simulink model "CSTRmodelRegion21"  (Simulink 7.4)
settings: Solver=ode15s  StartTime=0.0  StopTime=Tend  RelTol=1e-6
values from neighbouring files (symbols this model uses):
  cain = 2    [runDynSim321.m]    (also in sf_CSTR.m = cInVec(1))
  cbin = 1.5    [runDynSim321.m]    (also in sf_CSTR.m = cInVec(2))
undefined symbols (not defined in the file or in its folder): Floor, Ideal, internal, PI, Region2ControllerInitialValues, sigbuilder_block, Tdist, TimerScript, Tuninpars
libraries: simulink_extras x2

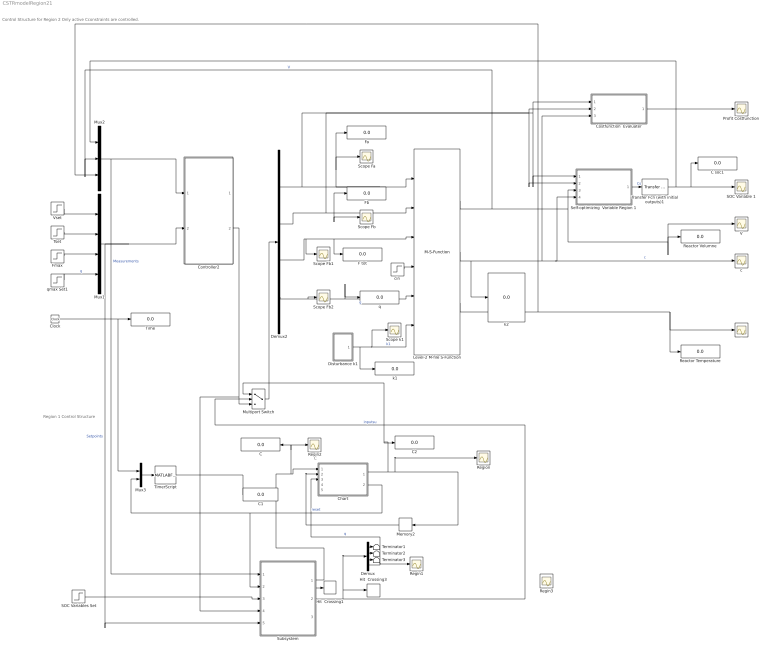
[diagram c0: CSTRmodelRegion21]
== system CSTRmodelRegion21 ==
  note: Control Structure for Region 2 Only active Cconstraints are controlled.
  note: Region 1 Control Structure
  note: C
  C : Display
  C soc1 : Display
  C1 : Display
  C2 : Display
  Chart : Stateflow chart
  Clock : Clock
  Controller2 : Subsystem
  Costfunction  Evaluater : Subsystem
  Demux : Demux
  Demux2 : Demux
  Disturbance k1 : Subsystem
  F tot : Display
  Fa : Display
  Fb : Display
  Fmax : Step  Time=0  Before=22  After=22  SampleTime=0
  Hit  Crossing1 : HitCross  HitCrossingOffset=1000  HitCrossingDirection=falling
  Hit  Crossing3 : HitCross  HitCrossingOffset=1000  HitCrossingDirection=rising
  Level-2 M-file S-Function : M-S-Function  FunctionName=sf_CSTR
  Memory2 : Memory  X0=1
  Multiport Switch : MultiPortSwitch  Inputs=2  OutDataType=fixdt(1, 16)  OutScaling=2^0
  Mux1 : Mux
  Mux2 : Mux  Inputs=3
  Mux3 : Mux  Inputs=2
  Profit Costfunction : Scope
  Reactor Temperature : Display
  Reactor Volumne : Display
  Regin1 : Scope
  Regin2 : Scope
  Regin3 : Scope
  Region : Scope
  SOC Variable 1 : Scope
  SOC Variables Set : Step  Time=0  After=0  SampleTime=0
  Scope Fa : Scope
  Scope Fb : Scope
  Scope Fb1 : Scope
  Scope Fb2 : Scope
  Scope k1 : Scope
  Self-optimizing  Variable Region 1 : Stateflow chart
  Subsystem : Subsystem
  T : Scope
  Terminator1 : Terminator
  Terminator2 : Terminator
  Terminator3 : Terminator
  Time : Display
  TimerScript : MATLABFcn  MATLABFcn=TimerScript(u(1),u(2))
  Transfer Fcn (with initial outputs)1 : simulink_extras/Additional Linear/Transfer Fcn (with initial outputs)  SystemSampleTime=-1  N=[1]  D="[1  1]"  Y0=41  U0=0
  Tset : Step  Time=250  Before=350  After=350  SampleTime=0
  V : Scope
  Vset : Step  Time=0  Before=500  After=500  SampleTime=0
  c : Scope
  cin : Step  Time=0  Before=[cain cbin 0 0]  After=[cain cbin 0 0]  SampleTime=0
  k1 : Display
  k2 : Display
  q : Display
  qmax Set1 : Step  Time=0  Before=1000  After=1000  SampleTime=0
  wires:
  cin/1 -> Level-2 M-file S-Function/4
  Level-2 M-file S-Function/1 -> Mux2/2, Self-optimizing  Variable Region 1/3(V), V/1, Reactor Volumne/1  "V"
  Level-2 M-file S-Function/2 -> Costfunction  Evaluater/3(Concentrations), c/1, Self-optimizing  Variable Region 1/4(cVector), k2/1  "c"
  Level-2 M-file S-Function/3 -> T/1, Reactor Temperature/1, Mux2/3  "T"
  Costfunction  Evaluater/1(Objective) -> Profit Costfunction/1
  Self-optimizing  Variable Region 1/1(cs) -> Transfer Fcn (with initial outputs)1/1  "Cs"
  Disturbance k1/1(Out1) -> Scope k1/1, Level-2 M-file S-Function/6, k1/1  "k1"
  Clock/1 -> Time/1, Mux3/1
  qmax Set1/1 -> Mux1/4  "q"
  Vset/1 -> Mux1/1
  Fmax/1 -> Mux1/3
  Tset/1 -> Mux1/2
  Mux2/1 -> Controller2/1(In1), Subsystem/1(In1)  "Measurements"
  Demux2/1 -> Costfunction  Evaluater/1(Fa), Self-optimizing  Variable Region 1/1(Fa), Level-2 M-file S-Function/1, Fa/1, Scope Fa/1
  Demux2/2 -> Costfunction  Evaluater/2(Fb), Self-optimizing  Variable Region 1/2(Fb), Scope Fb/1, Level-2 M-file S-Function/2, Fb/1
  Demux2/3 -> Level-2 M-file S-Function/3, F tot/1, Scope Fb1/1
  Demux2/4 -> Level-2 M-file S-Function/5, q/1, Scope Fb2/1  "q"
  Mux1/1 -> Controller2/2(In2), Subsystem/5(In5)  "Setpoints"
  Controller2/2(Out6) -> Multiport Switch/3, Subsystem/4(In4)
  SOC Variables Set/1 -> Subsystem/3(In3)
  Chart/2(reset) -> Subsystem/2(In2), Mux3/2  "reset"
  Multiport Switch/1 -> Demux2/1
  Subsystem/2(Out2) -> Hit  Crossing3/1, Demux/1, Multiport Switch/2  "inputsu"
  Transfer Fcn (with initial outputs)1/1 -> Mux2/1, SOC Variable 1/1, C soc1/1
  Subsystem/1(Out1) -> Chart/1(c1), C/1, Regin2/1, Hit  Crossing1/1
  Mux3/1 -> TimerScript/1
  TimerScript/1 -> C1/1
  Memory2/1 -> Chart/2(r)
  Demux/1 -> Terminator1/1
  Demux/2 -> Terminator2/1
  Demux/3 -> Terminator3/1
  Demux/4 -> Chart/3(q), Regin1/1  "q"
  Chart/1(R) -> Region/1, Memory2/1, C2/1, Multiport Switch/1

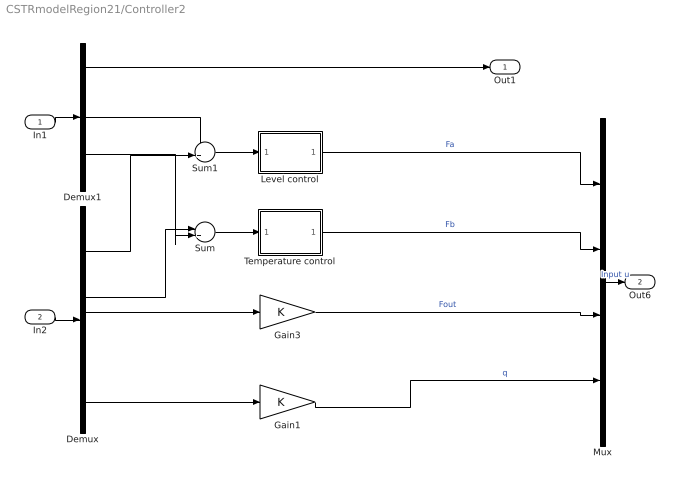
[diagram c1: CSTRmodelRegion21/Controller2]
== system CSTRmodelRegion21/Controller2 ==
  In1 : Inport
  In2 : Inport  Port=2
  Demux : Demux
  Demux1 : Demux  Outputs=3
  Gain1 : Gain  ParameterDataType=fixdt(1, 16)  ParameterScaling=2^0  OutDataType=fixdt(1, 16)  OutScaling=2^0
  Gain3 : Gain  ParameterDataType=fixdt(1, 16)  ParameterScaling=2^0  OutDataType=fixdt(1, 16)  OutScaling=2^0
  Level control : Subsystem  AncestorBlock=simulink/Continuous/PID Controller  DialogController=pidpack.PIDConfig.pidDDGCreate  DialogControllerArgs=DataTag0  mask(PID 1dof){Controller=PI, TimeDomain=Continuous-time, SampleTime=1, IntegratorMethod=Forward Euler, FilterMethod=Forward Euler, Form=Ideal, P=35*2, I=0.024, D=0, N=100, InitialConditionSource=internal, InitialConditionForIntegrator=Region2ControllerInitialValues.Level, InitialConditionForFilter=0, ExternalReset=none, IgnoreLimit=off, ZeroCross=on, LimitOutput=on, UpperSaturationLimit=10, LowerSaturationLimit=4, LinearizeAsGain=off, AntiWindupMode=back-calculation, Kb=1, TrackingMode=off, Kt=1, RndMeth=Floor, SaturateOnIntegerOverflow=off, LockScale=off, PParamMin=[], PParamMax=[], PParamDataTypeStr=Inherit: Inherit via internal rule, IParamMin=[], IParamMax=[], IParamDataTypeStr=Inherit: Inherit via internal rule, DParamMin=[], DParamMax=[], DParamDataTypeStr=Inherit: Inherit via internal rule, NParamMin=[], NParamMax=[], NParamDataTypeStr=Inherit: Inherit via internal rule, KbParamMin=[], KbParamMax=[], KbParamDataTypeStr=Inherit: Inherit via internal rule, KtParamMin=[], KtParamMax=[], KtParamDataTypeStr=Inherit: Inherit via internal rule, POutMin=[], POutMax=[], POutDataTypeStr=Inherit: Inherit via internal rule, IOutMin=[], IOutMax=[], IOutDataTypeStr=Inherit: Inherit via internal rule, DOutMin=[], DOutMax=[], DOutDataTypeStr=Inherit: Inherit via internal rule, NOutMin=[], NOutMax=[], NOutDataTypeStr=Inherit: Inherit via internal rule, KbOutMin=[], KbOutMax=[], KbOutDataTypeStr=Inherit: Inherit via internal rule, KtOutMin=[], KtOutMax=[], KtOutDataTypeStr=Inherit: Inherit via internal rule, IntegratorOutMin=[], IntegratorOutMax=[], IntegratorOutDataTypeStr=Inherit: Inherit via internal rule, FilterOutMin=[], FilterOutMax=[], FilterOutDataTypeStr=Inherit: Inherit via internal rule, SumOutMin=[], SumOutMax=[], SumOutDataTypeStr=Inherit: Inherit via internal rule, SumI1OutMin=[], SumI1OutMax=[], SumI1OutDataTypeStr=Inherit: Inherit via internal rule, SumI2OutMin=[], SumI2OutMax=[], SumI2OutDataTypeStr=Inherit: Inherit via internal rule, SumI3OutMin=[], SumI3OutMax=[], SumI3OutDataTypeStr=Inherit: Inherit via internal rule, SumDOutMin=[], SumDOutMax=[], SumDOutDataTypeStr=Inherit: Inherit via internal rule, SumAccumDataTypeStr=Inherit: Inherit via internal rule, SumI1AccumDataTypeStr=Inherit: Inherit via internal rule, SumI2AccumDataTypeStr=Inherit: Inherit via internal rule, SumI3AccumDataTypeStr=Inherit: Inherit via internal rule, SumDAccumDataTypeStr=Inherit: Inherit via internal rule, SaturationOutMin=[], SaturationOutMax=[], SaturationOutDataTypeStr=Inherit: Same as input, IntegratorContinuousStateAttributes='', IntegratorStateIdentifier=, IntegratorStateMustResolveToSignalObject=off, IntegratorRTWStateStorageClass=Auto, IntegratorRTWStateStorageTypeQualifier=, FilterContinuousStateAttributes='', FilterStateIdentifier=, FilterStateMustResolveToSignalObject=off, FilterRTWStateStorageClass=Auto, FilterRTWStateStorageTypeQualifier=}
      mask prompts: TimeDomain "Time-domain:"; SampleTime "Sample time (-1 for inherited):"; IntegratorMethod "Integrator method:"; FilterMethod "Filter method:"; Form "Controller form:"; P "Proportional (P):"; I "Integral (I):"; D "Derivative (D):"; N "Filter coefficient (N):"; InitialConditionSource "Source:"; InitialConditionForIntegrator "Integrator:"; InitialConditionForFilter "Filter:"; ExternalReset "External reset:"; IgnoreLimit "Ignore reset when linearizing"; ZeroCross "Enable zero-crossing detection"; LimitOutput "Limit output"; UpperSaturationLimit "Upper saturation limit:"; LowerSaturationLimit "Lower saturation limit:"; LinearizeAsGain "Ignore saturation when linearizing"; AntiWindupMode "Anti-windup method:"; Kb "Back-calculation coefficient (Kb):"; TrackingMode "Enable tracking mode"; Kt "Tracking coefficient (Kt):"; RndMeth "Integer rounding mode:"; SaturateOnIntegerOverflow "Saturate on integer overflow"; LockScale "Lock data type settings against changes by the fixed-point tools"; PParamMin "P parameter minimum:"; PParamMax "P parameter maximum:"; PParamDataTypeStr "P parameter:"; IParamMin "I parameter minimum:"; IParamMax "I parameter maximum:"; IParamDataTypeStr "I parameter:"; DParamMin "D parameter minimum:"; DParamMax "D parameter maximum:"; DParamDataTypeStr "D parameter:"; NParamMin "N parameter minimum:"; NParamMax "N parameter maximum:"; NParamDataTypeStr "N parameter:"; KbParamMin "Kb parameter minimum:"; KbParamMax "Kb parameter maximum:"; KbParamDataTypeStr "Kb parameter:"; KtParamMin "Kt parameter minimum:"; KtParamMax "Kt parameter maximum:"; KtParamDataTypeStr "Kt parameter:"; POutMin "P product output minimum:"; POutMax "P product output maximum:"; POutDataTypeStr "P product output:"; IOutMin "I product output minimum:"; IOutMax "I product output maximum:"; IOutDataTypeStr "I product output:"; DOutMin "D product output minimum:"; DOutMax "D product output maximum:"; DOutDataTypeStr "D product output:"; NOutMin "N product output minimum:"; NOutMax "N product output maximum:"; NOutDataTypeStr "N product output:"; KbOutMin "Kb product output minimum:"; KbOutMax "Kb product output maximum:"; KbOutDataTypeStr "Kb product output:"; KtOutMin "Kt product output minimum:"; KtOutMax "Kt product output maximum:"; KtOutDataTypeStr "Kt product output:"; IntegratorOutMin "Integrator output minimum:"; IntegratorOutMax "Integrator output maximum:"; IntegratorOutDataTypeStr "Integrator output:"; FilterOutMin "Filter output minimum:"; FilterOutMax "Filter output maximum:"; FilterOutDataTypeStr "Filter output:"; SumOutMin "Sum output minimum:"; SumOutMax "Sum output maximum:"; SumOutDataTypeStr "Sum output:"; SumI1OutMin "SumI1 output minimum:"; SumI1OutMax "SumI1 output maximum:"; SumI1OutDataTypeStr "SumI1 output:"; SumI2OutMin "SumI2 output minimum:"; SumI2OutMax "SumI2 output maximum:"; SumI2OutDataTypeStr "SumI2 output:"; SumI3OutMin "SumI3 output minimum:"; SumI3OutMax "SumI3 output maximum:"; SumI3OutDataTypeStr "SumI3 output:"; SumDOutMin "SumD output minimum:"; SumDOutMax "SumD output maximum:"; SumDOutDataTypeStr "SumD output:"; SumAccumDataTypeStr "Accumulator of Sum:"; SumI1AccumDataTypeStr "Accumulator of SumI1:"; SumI2AccumDataTypeStr "Accumulator of SumI2:"; SumI3AccumDataTypeStr "Accumulator of SumI3:"; SumDAccumDataTypeStr "Accumulator of SumD:"; SaturationOutMin "Saturation output minimum:"; SaturationOutMax "Saturation output maximum:"; SaturationOutDataTypeStr "Saturation output:"; IntegratorContinuousStateAttributes "State name: (e.g., 'position')"; IntegratorStateIdentifier "State name:"; IntegratorStateMustResolveToSignalObject "State name must resolve to Simulink signal object"; IntegratorRTWStateStorageClass "Real-Time Workshop storage class:"; IntegratorRTWStateStorageTypeQualifier "Real-Time Workshop storage type qualifier:"; FilterContinuousStateAttributes "State name: (e.g., 'position')"; FilterStateIdentifier "State name:"; FilterStateMustResolveToSignalObject "State name must resolve to Simulink signal object"; FilterRTWStateStorageClass "Real-Time Workshop storage class:"; FilterRTWStateStorageTypeQualifier "Real-Time Workshop storage type qualifier:"
      mask help: This block implements continuous- and discrete-time PID control algorithms and includes advanced features such as anti-windup, external reset, and signal tracking. You can tune the PID gains automatically using the 'Tune...' button (requires Simulink Control Design).
      mask init:
      | [shiftx shifty satshiftx satshifty] = pidpack.PIDConfig.configPID(gcbh);
  Mux : Mux
  Sum : Sum  Inputs=|+-  OutDataType=fixdt(1, 16)  OutScaling=2^0
  Sum1 : Sum  Inputs=-+|  OutDataType=fixdt(1, 16)  OutScaling=2^0
  Temperature control : Subsystem  AncestorBlock=simulink/Continuous/PID Controller  DialogController=pidpack.PIDConfig.pidDDGCreate  DialogControllerArgs=DataTag1  mask(PID 1dof){Controller=PI, TimeDomain=Continuous-time, SampleTime=1, IntegratorMethod=Forward Euler, FilterMethod=Forward Euler, Form=Ideal, P=-0.845/2/5, I=1, D=0, N=100, InitialConditionSource=internal, InitialConditionForIntegrator=Region2ControllerInitialValues.Temperature, InitialConditionForFilter=0, ExternalReset=none, IgnoreLimit=off, ZeroCross=on, LimitOutput=on, UpperSaturationLimit=1e3, LowerSaturationLimit=10, LinearizeAsGain=off, AntiWindupMode=back-calculation, Kb=1, TrackingMode=off, Kt=1, RndMeth=Floor, SaturateOnIntegerOverflow=off, LockScale=off, PParamMin=[], PParamMax=[], PParamDataTypeStr=Inherit: Inherit via internal rule, IParamMin=[], IParamMax=[], IParamDataTypeStr=Inherit: Inherit via internal rule, DParamMin=[], DParamMax=[], DParamDataTypeStr=Inherit: Inherit via internal rule, NParamMin=[], NParamMax=[], NParamDataTypeStr=Inherit: Inherit via internal rule, KbParamMin=[], KbParamMax=[], KbParamDataTypeStr=Inherit: Inherit via internal rule, KtParamMin=[], KtParamMax=[], KtParamDataTypeStr=Inherit: Inherit via internal rule, POutMin=[], POutMax=[], POutDataTypeStr=Inherit: Inherit via internal rule, IOutMin=[], IOutMax=[], IOutDataTypeStr=Inherit: Inherit via internal rule, DOutMin=[], DOutMax=[], DOutDataTypeStr=Inherit: Inherit via internal rule, NOutMin=[], NOutMax=[], NOutDataTypeStr=Inherit: Inherit via internal rule, KbOutMin=[], KbOutMax=[], KbOutDataTypeStr=Inherit: Inherit via internal rule, KtOutMin=[], KtOutMax=[], KtOutDataTypeStr=Inherit: Inherit via internal rule, IntegratorOutMin=[], IntegratorOutMax=[], IntegratorOutDataTypeStr=Inherit: Inherit via internal rule, FilterOutMin=[], FilterOutMax=[], FilterOutDataTypeStr=Inherit: Inherit via internal rule, SumOutMin=[], SumOutMax=[], SumOutDataTypeStr=Inherit: Inherit via internal rule, SumI1OutMin=[], SumI1OutMax=[], SumI1OutDataTypeStr=Inherit: Inherit via internal rule, SumI2OutMin=[], SumI2OutMax=[], SumI2OutDataTypeStr=Inherit: Inherit via internal rule, SumI3OutMin=[], SumI3OutMax=[], SumI3OutDataTypeStr=Inherit: Inherit via internal rule, SumDOutMin=[], SumDOutMax=[], SumDOutDataTypeStr=Inherit: Inherit via internal rule, SumAccumDataTypeStr=Inherit: Inherit via internal rule, SumI1AccumDataTypeStr=Inherit: Inherit via internal rule, SumI2AccumDataTypeStr=Inherit: Inherit via internal rule, SumI3AccumDataTypeStr=Inherit: Inherit via internal rule, SumDAccumDataTypeStr=Inherit: Inherit via internal rule, SaturationOutMin=[], SaturationOutMax=[], SaturationOutDataTypeStr=Inherit: Same as input, IntegratorContinuousStateAttributes='', IntegratorStateIdentifier=, IntegratorStateMustResolveToSignalObject=off, IntegratorRTWStateStorageClass=Auto, IntegratorRTWStateStorageTypeQualifier=, FilterContinuousStateAttributes='', FilterStateIdentifier=, FilterStateMustResolveToSignalObject=off, FilterRTWStateStorageClass=Auto, FilterRTWStateStorageTypeQualifier=}
      mask prompts: TimeDomain "Time-domain:"; SampleTime "Sample time (-1 for inherited):"; IntegratorMethod "Integrator method:"; FilterMethod "Filter method:"; Form "Controller form:"; P "Proportional (P):"; I "Integral (I):"; D "Derivative (D):"; N "Filter coefficient (N):"; InitialConditionSource "Source:"; InitialConditionForIntegrator "Integrator:"; InitialConditionForFilter "Filter:"; ExternalReset "External reset:"; IgnoreLimit "Ignore reset when linearizing"; ZeroCross "Enable zero-crossing detection"; LimitOutput "Limit output"; UpperSaturationLimit "Upper saturation limit:"; LowerSaturationLimit "Lower saturation limit:"; LinearizeAsGain "Ignore saturation when linearizing"; AntiWindupMode "Anti-windup method:"; Kb "Back-calculation coefficient (Kb):"; TrackingMode "Enable tracking mode"; Kt "Tracking coefficient (Kt):"; RndMeth "Integer rounding mode:"; SaturateOnIntegerOverflow "Saturate on integer overflow"; LockScale "Lock data type settings against changes by the fixed-point tools"; PParamMin "P parameter minimum:"; PParamMax "P parameter maximum:"; PParamDataTypeStr "P parameter:"; IParamMin "I parameter minimum:"; IParamMax "I parameter maximum:"; IParamDataTypeStr "I parameter:"; DParamMin "D parameter minimum:"; DParamMax "D parameter maximum:"; DParamDataTypeStr "D parameter:"; NParamMin "N parameter minimum:"; NParamMax "N parameter maximum:"; NParamDataTypeStr "N parameter:"; KbParamMin "Kb parameter minimum:"; KbParamMax "Kb parameter maximum:"; KbParamDataTypeStr "Kb parameter:"; KtParamMin "Kt parameter minimum:"; KtParamMax "Kt parameter maximum:"; KtParamDataTypeStr "Kt parameter:"; POutMin "P product output minimum:"; POutMax "P product output maximum:"; POutDataTypeStr "P product output:"; IOutMin "I product output minimum:"; IOutMax "I product output maximum:"; IOutDataTypeStr "I product output:"; DOutMin "D product output minimum:"; DOutMax "D product output maximum:"; DOutDataTypeStr "D product output:"; NOutMin "N product output minimum:"; NOutMax "N product output maximum:"; NOutDataTypeStr "N product output:"; KbOutMin "Kb product output minimum:"; KbOutMax "Kb product output maximum:"; KbOutDataTypeStr "Kb product output:"; KtOutMin "Kt product output minimum:"; KtOutMax "Kt product output maximum:"; KtOutDataTypeStr "Kt product output:"; IntegratorOutMin "Integrator output minimum:"; IntegratorOutMax "Integrator output maximum:"; IntegratorOutDataTypeStr "Integrator output:"; FilterOutMin "Filter output minimum:"; FilterOutMax "Filter output maximum:"; FilterOutDataTypeStr "Filter output:"; SumOutMin "Sum output minimum:"; SumOutMax "Sum output maximum:"; SumOutDataTypeStr "Sum output:"; SumI1OutMin "SumI1 output minimum:"; SumI1OutMax "SumI1 output maximum:"; SumI1OutDataTypeStr "SumI1 output:"; SumI2OutMin "SumI2 output minimum:"; SumI2OutMax "SumI2 output maximum:"; SumI2OutDataTypeStr "SumI2 output:"; SumI3OutMin "SumI3 output minimum:"; SumI3OutMax "SumI3 output maximum:"; SumI3OutDataTypeStr "SumI3 output:"; SumDOutMin "SumD output minimum:"; SumDOutMax "SumD output maximum:"; SumDOutDataTypeStr "SumD output:"; SumAccumDataTypeStr "Accumulator of Sum:"; SumI1AccumDataTypeStr "Accumulator of SumI1:"; SumI2AccumDataTypeStr "Accumulator of SumI2:"; SumI3AccumDataTypeStr "Accumulator of SumI3:"; SumDAccumDataTypeStr "Accumulator of SumD:"; SaturationOutMin "Saturation output minimum:"; SaturationOutMax "Saturation output maximum:"; SaturationOutDataTypeStr "Saturation output:"; IntegratorContinuousStateAttributes "State name: (e.g., 'position')"; IntegratorStateIdentifier "State name:"; IntegratorStateMustResolveToSignalObject "State name must resolve to Simulink signal object"; IntegratorRTWStateStorageClass "Real-Time Workshop storage class:"; IntegratorRTWStateStorageTypeQualifier "Real-Time Workshop storage type qualifier:"; FilterContinuousStateAttributes "State name: (e.g., 'position')"; FilterStateIdentifier "State name:"; FilterStateMustResolveToSignalObject "State name must resolve to Simulink signal object"; FilterRTWStateStorageClass "Real-Time Workshop storage class:"; FilterRTWStateStorageTypeQualifier "Real-Time Workshop storage type qualifier:"
      mask help: This block implements continuous- and discrete-time PID control algorithms and includes advanced features such as anti-windup, external reset, and signal tracking. You can tune the PID gains automatically using the 'Tune...' button (requires Simulink Control Design).
      mask init:
      | [shiftx shifty satshiftx satshifty] = pidpack.PIDConfig.configPID(gcbh);
  Out1 : Outport
  Out6 : Outport  Port=2
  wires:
  Sum/1 -> Temperature control/1(u)
  Sum1/1 -> Level control/1(u)
  Demux/1 -> Sum1/2
  Demux/2 -> Sum/1
  Demux/3 -> Gain3/1
  Demux/4 -> Gain1/1
  Demux1/2 -> Sum1/1
  Demux1/3 -> Sum/2
  Demux1/1 -> Out1/1
  In1/1 -> Demux1/1
  Level control/1(y) -> Mux/1  "Fa"
  Temperature control/1(y) -> Mux/2  "Fb"
  Gain3/1 -> Mux/3  "Fout"
  In2/1 -> Demux/1
  Gain1/1 -> Mux/4  "q"
  Mux/1 -> Out6/1  "Input u"

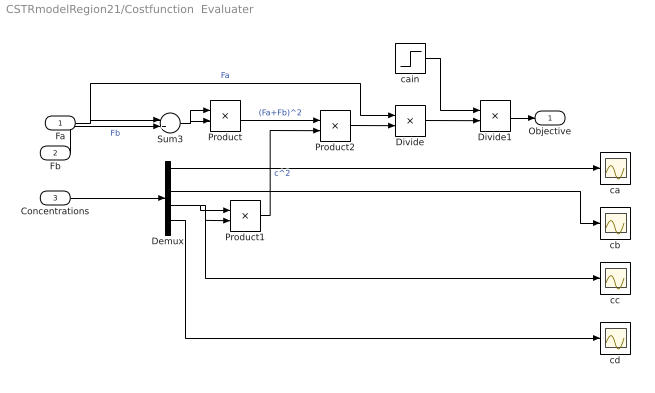
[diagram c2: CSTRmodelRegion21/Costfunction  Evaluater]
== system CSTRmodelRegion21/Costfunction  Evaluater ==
  Fa : Inport
  Fb : Inport  Port=2
  Concentrations : Inport  Port=3
  Demux : Demux
  Divide : Product  Inputs=/*  OutDataType=fixdt(1, 16)  OutScaling=2^-10
  Divide1 : Product  Inputs=/*  OutDataType=fixdt(1, 16)  OutScaling=2^-10
  Product : Product  OutDataType=fixdt(1, 16)  OutScaling=2^0
  Product1 : Product  OutDataType=fixdt(1, 16)  OutScaling=2^0
  Product2 : Product  OutDataType=fixdt(1, 16)  OutScaling=2^0
  Sum3 : Sum  Inputs=|++  OutDataType=fixdt(1, 16)  OutScaling=2^0
  ca : Scope
  cain : Step  Before=cain  After=cain  SampleTime=0
  cb : Scope
  cc : Scope
  cd : Scope
  Objective : Outport
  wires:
  Sum3/1 -> Product/1, Product/2
  Demux/3 -> Product1/1, Product1/2, cc/1
  Product/1 -> Product2/1  "(Fa+Fb)^2"
  Product1/1 -> Product2/2  "c^2"
  Product2/1 -> Divide/2
  Divide/1 -> Divide1/2
  cain/1 -> Divide1/1
  Fa/1 -> Sum3/1, Divide/1  "Fa"
  Fb/1 -> Sum3/2  "Fb"
  Concentrations/1 -> Demux/1
  Divide1/1 -> Objective/1
  Demux/1 -> ca/1
  Demux/2 -> cb/1
  Demux/4 -> cd/1

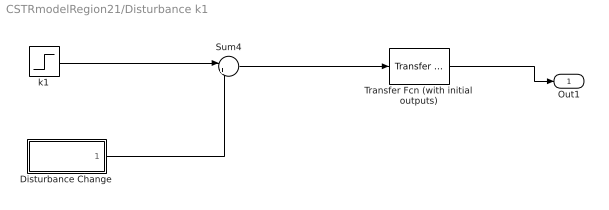
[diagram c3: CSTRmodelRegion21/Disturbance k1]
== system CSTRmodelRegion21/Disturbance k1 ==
  Disturbance Change : Subsystem  Tag=STV Subsys  LoadFcn=sigbuilder_block('load');  StartFcn=sigbuilder_block('start');  StopFcn=sigbuilder_block('stop');  ClipboardFcn=sigbuilder_block('clipboard');
  Sum4 : Sum  Inputs=|++  OutDataType=fixdt(1, 16)  OutScaling=2^0
  Transfer Fcn (with initial outputs) : simulink_extras/Additional Linear/Transfer Fcn (with initial outputs)  SystemSampleTime=-1  N=[1]  D="[50  1]"  Y0=0.75  U0=0
  k1 : Step  Time=Tdist  After=0  SampleTime=0
  Out1 : Outport
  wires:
  Sum4/1 -> Transfer Fcn (with initial outputs)/1
  Disturbance Change/1(Signal 1) -> Sum4/2
  k1/1 -> Sum4/1
  Transfer Fcn (with initial outputs)/1 -> Out1/1

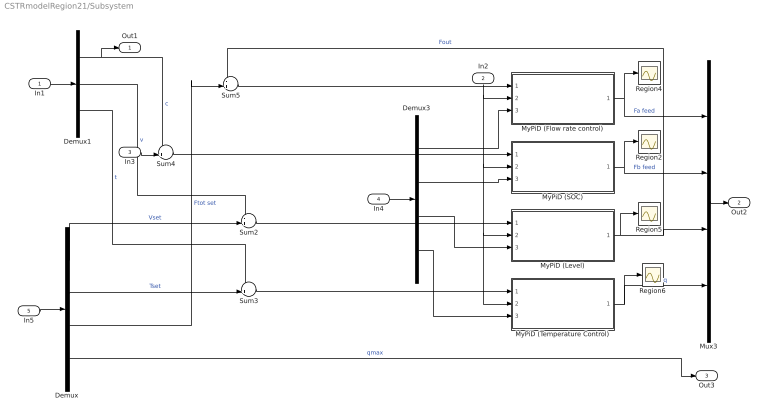
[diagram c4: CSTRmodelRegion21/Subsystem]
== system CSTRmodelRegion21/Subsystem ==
  In1 : Inport
  In2 : Inport  Port=2
  In3 : Inport  Port=3
  In4 : Inport  Port=4
  In5 : Inport  Port=5
  Demux : Demux
  Demux1 : Demux  Outputs=3
  Demux3 : Demux
  Mux3 : Mux
  MyPiD (Flow rate control) : Subsystem  mask{Kp=Tuninpars.Reg1.FlowController.Kp, TauiInv=Tuninpars.Reg1.FlowController.TauiInv, UB=[inf], LB=2}
      mask prompts: Kp "Proportional Gain Kp"; TauiInv "Inverse Integral time"; UB "Upper bound"; LB "Lower bound"
  MyPiD (Level) : Subsystem  mask{Kp=Tuninpars.Reg1.LevelController.Kp, TauiInv=Tuninpars.Reg1.LevelController.TauiInv, UB=[40], LB=2}
      mask prompts: Kp "Proportional Gain Kp"; TauiInv "Inverse Integral time"; UB "Upper bound"; LB "Lower bound"
  MyPiD (SOC) : Subsystem  mask{Kp=Tuninpars.Reg1.SocController.Kp, TauiInv=Tuninpars.Reg1.SocController.TauiInv, UB=inf, LB=2}
      mask prompts: Kp "Proportional Gain Kp"; TauiInv "Inverse Integral time"; UB "Upper bound"; LB "Lower bound"
  MyPiD (Temperature Control) : Subsystem  mask{Kp=Tuninpars.Reg1.TempController.Kp, TauiInv=Tuninpars.Reg1.TempController.TauiInv, UB=1000, LB=1}
      mask prompts: Kp "Proportional Gain Kp"; TauiInv "Inverse Integral time"; UB "Upper bound"; LB "Lower bound"
  Region{2,4..6} (4 alike) : Scope
  Sum{2..5} (4 alike) : Sum  Inputs=-+|  OutDataType=fixdt(1, 16)  OutScaling=2^0
  Out1 : Outport
  Out2 : Outport  Port=2
  Out3 : Outport  Port=3
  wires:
  Sum5/1 -> MyPiD (Flow rate control)/1(In1)
  Sum4/1 -> MyPiD (SOC)/1(In1)
  MyPiD (SOC)/1(Out1) -> Mux3/2, Region2/1  "Fb feed"
  Sum2/1 -> MyPiD (Level)/1(In1)
  MyPiD (Level)/1(Out1) -> Sum5/1, Mux3/3, Region5/1  "Fout"
  Sum3/1 -> MyPiD (Temperature Control)/1(In1)
  MyPiD (Temperature Control)/1(Out1) -> Region6/1, Mux3/4  "q"
  Demux1/1 -> Sum4/1, Out1/1  "c"
  Demux1/2 -> Sum2/1  "v"
  Demux1/3 -> Sum3/1  "t"
  Demux/3 -> Sum5/2  "Ftot set"
  MyPiD (Flow rate control)/1(Out1) -> Mux3/1, Region4/1  "Fa feed"
  Demux/2 -> Sum3/2  "Tset"
  Demux/1 -> Sum2/2  "Vset"
  Demux3/1 -> MyPiD (Flow rate control)/3(In3)
  Demux3/2 -> MyPiD (SOC)/3(In3)
  Demux3/3 -> MyPiD (Level)/3(In3)
  Demux3/4 -> MyPiD (Temperature Control)/3(In3)
  In1/1 -> Demux1/1
  In2/1 -> MyPiD (Flow rate control)/2(In2), MyPiD (SOC)/2(In2), MyPiD (Temperature Control)/2(In2), MyPiD (Level)/2(In2)
  In4/1 -> Demux3/1
  In5/1 -> Demux/1
  In3/1 -> Sum4/2
  Mux3/1 -> Out2/1
  Demux/4 -> Out3/1  "qmax"

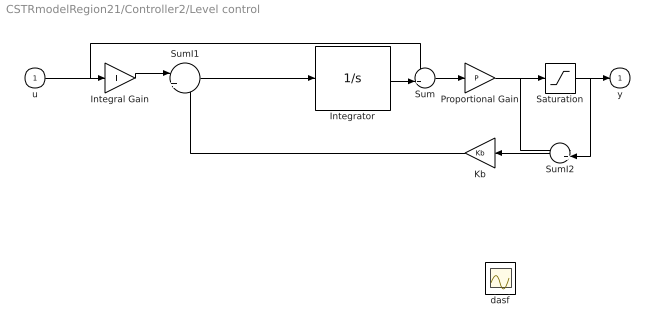
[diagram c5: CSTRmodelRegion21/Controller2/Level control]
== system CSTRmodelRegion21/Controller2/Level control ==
  u : Inport  OutDataType=OutDataTypeStr
  Integral Gain : Gain  DisableCoverage=on  Gain=I  ParamMin=IParamMin  ParamMax=IParamMax  ParameterDataTypeMode=Specify via dialog  ParameterDataType=IParamDataTypeStr  ParamDataTypeStr=IParamDataTypeStr  OutMin=IOutMin  OutMax=IOutMax  OutDataTypeMode=Specify via dialog  OutDataType=IOutDataTypeStr  OutDataTypeStr=IOutDataTypeStr
  Integrator : Integrator  DisableCoverage=on  InitialCondition=InitialConditionForIntegrator
  Kb : Gain  DisableCoverage=on  Gain=Kb  ParamMin=KbParamMin  ParamMax=KbParamMax  ParameterDataTypeMode=Specify via dialog  ParameterDataType=KbParamDataTypeStr  ParamDataTypeStr=KbParamDataTypeStr  OutMin=KbOutMin  OutMax=KbOutMax  OutDataTypeMode=Specify via dialog  OutDataType=KbOutDataTypeStr  OutDataTypeStr=KbOutDataTypeStr
  Proportional Gain : Gain  DisableCoverage=on  Gain=P  ParamMin=PParamMin  ParamMax=PParamMax  ParameterDataTypeMode=Specify via dialog  ParameterDataType=PParamDataTypeStr  ParamDataTypeStr=PParamDataTypeStr  OutMin=POutMin  OutMax=POutMax  OutDataTypeMode=Specify via dialog  OutDataType=POutDataTypeStr  OutDataTypeStr=POutDataTypeStr
  Saturation : Saturate  UpperLimit=UpperSaturationLimit  LowerLimit=LowerSaturationLimit  LinearizeAsGain=off  OutMin=SaturationOutMin  OutMax=SaturationOutMax  OutDataTypeMode=Specify via dialog  OutDataType=SaturationOutDataTypeStr  OutDataTypeStr=SaturationOutDataTypeStr
  Sum : Sum  DisableCoverage=on  Inputs=++|  AccumDataTypeStr=SumAccumDataTypeStr  OutMin=SumOutMin  OutMax=SumOutMax  OutDataTypeMode=Specify via dialog  OutDataType=SumOutDataTypeStr  OutDataTypeStr=SumOutDataTypeStr
  SumI1 : Sum  DisableCoverage=on  Inputs=|++  AccumDataTypeStr=SumI1AccumDataTypeStr  OutMin=SumI1OutMin  OutMax=SumI1OutMax  OutDataTypeMode=Specify via dialog  OutDataType=SumI1OutDataTypeStr  OutDataTypeStr=SumI1OutDataTypeStr
  SumI2 : Sum  DisableCoverage=on  Inputs=-+|  AccumDataTypeStr=SumI2AccumDataTypeStr  OutMin=SumI2OutMin  OutMax=SumI2OutMax  OutDataTypeMode=Specify via dialog  OutDataType=SumI2OutDataTypeStr  OutDataTypeStr=SumI2OutDataTypeStr
  dasf : Scope
  y : Outport  OutDataType=OutDataTypeStr  InitialOutput=0
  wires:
  u/1 -> Sum/1, Integral Gain/1
  Integrator/1 -> Sum/2
  Sum/1 -> Proportional Gain/1
  Saturation/1 -> y/1, SumI2/2
  Proportional Gain/1 -> Saturation/1, SumI2/1
  SumI2/1 -> Kb/1
  Kb/1 -> SumI1/2
  SumI1/1 -> Integrator/1
  Integral Gain/1 -> SumI1/1

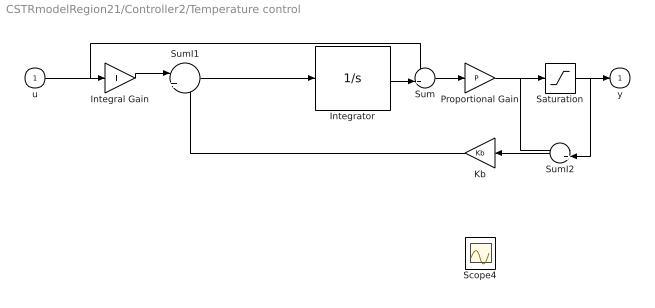
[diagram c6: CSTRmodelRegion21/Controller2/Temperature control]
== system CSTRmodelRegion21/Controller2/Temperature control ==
  u : Inport  OutDataType=OutDataTypeStr
  Integral Gain : Gain  DisableCoverage=on  Gain=I  ParamMin=IParamMin  ParamMax=IParamMax  ParameterDataTypeMode=Specify via dialog  ParameterDataType=IParamDataTypeStr  ParamDataTypeStr=IParamDataTypeStr  OutMin=IOutMin  OutMax=IOutMax  OutDataTypeMode=Specify via dialog  OutDataType=IOutDataTypeStr  OutDataTypeStr=IOutDataTypeStr
  Integrator : Integrator  DisableCoverage=on  InitialCondition=InitialConditionForIntegrator
  Kb : Gain  DisableCoverage=on  Gain=Kb  ParamMin=KbParamMin  ParamMax=KbParamMax  ParameterDataTypeMode=Specify via dialog  ParameterDataType=KbParamDataTypeStr  ParamDataTypeStr=KbParamDataTypeStr  OutMin=KbOutMin  OutMax=KbOutMax  OutDataTypeMode=Specify via dialog  OutDataType=KbOutDataTypeStr  OutDataTypeStr=KbOutDataTypeStr
  Proportional Gain : Gain  DisableCoverage=on  Gain=P  ParamMin=PParamMin  ParamMax=PParamMax  ParameterDataTypeMode=Specify via dialog  ParameterDataType=PParamDataTypeStr  ParamDataTypeStr=PParamDataTypeStr  OutMin=POutMin  OutMax=POutMax  OutDataTypeMode=Specify via dialog  OutDataType=POutDataTypeStr  OutDataTypeStr=POutDataTypeStr
  Saturation : Saturate  UpperLimit=UpperSaturationLimit  LowerLimit=LowerSaturationLimit  LinearizeAsGain=off  OutMin=SaturationOutMin  OutMax=SaturationOutMax  OutDataTypeMode=Specify via dialog  OutDataType=SaturationOutDataTypeStr  OutDataTypeStr=SaturationOutDataTypeStr
  Scope4 : Scope
  Sum : Sum  DisableCoverage=on  Inputs=++|  AccumDataTypeStr=SumAccumDataTypeStr  OutMin=SumOutMin  OutMax=SumOutMax  OutDataTypeMode=Specify via dialog  OutDataType=SumOutDataTypeStr  OutDataTypeStr=SumOutDataTypeStr
  SumI1 : Sum  DisableCoverage=on  Inputs=|++  AccumDataTypeStr=SumI1AccumDataTypeStr  OutMin=SumI1OutMin  OutMax=SumI1OutMax  OutDataTypeMode=Specify via dialog  OutDataType=SumI1OutDataTypeStr  OutDataTypeStr=SumI1OutDataTypeStr
  SumI2 : Sum  DisableCoverage=on  Inputs=-+|  AccumDataTypeStr=SumI2AccumDataTypeStr  OutMin=SumI2OutMin  OutMax=SumI2OutMax  OutDataTypeMode=Specify via dialog  OutDataType=SumI2OutDataTypeStr  OutDataTypeStr=SumI2OutDataTypeStr
  y : Outport  OutDataType=OutDataTypeStr  InitialOutput=0
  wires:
  u/1 -> Sum/1, Integral Gain/1
  Integrator/1 -> Sum/2
  Sum/1 -> Proportional Gain/1
  Saturation/1 -> y/1, SumI2/2
  Proportional Gain/1 -> Saturation/1, SumI2/1
  SumI2/1 -> Kb/1
  Kb/1 -> SumI1/2
  SumI1/1 -> Integrator/1
  Integral Gain/1 -> SumI1/1

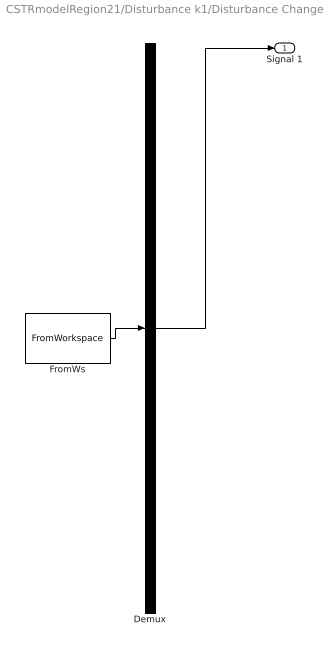
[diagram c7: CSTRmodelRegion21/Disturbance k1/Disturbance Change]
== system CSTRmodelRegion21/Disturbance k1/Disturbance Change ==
  Demux : Demux  Tag=STV Demux  Outputs=1
  FromWs : FromWorkspace  Tag=STV FromWs  VariableName=tuvar  SampleTime=0  SigBuilderData=DataTag2  VnvData=DataTag3
  Signal 1 : Outport  Tag=STV Outport  OutDataType=fixdt(1, 16)  OutScaling=2^0
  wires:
  FromWs/1 -> Demux/1
  Demux/1 -> Signal 1/1

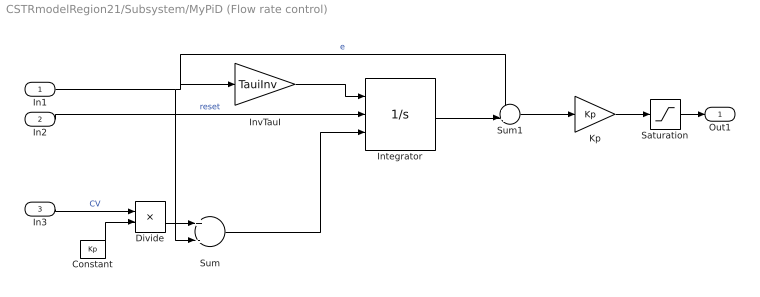
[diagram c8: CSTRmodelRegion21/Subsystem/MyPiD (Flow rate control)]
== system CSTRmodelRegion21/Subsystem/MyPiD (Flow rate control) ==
  In1 : Inport
  In2 : Inport  Port=2
  In3 : Inport  Port=3
  Constant : Constant  Value=Kp  OutDataType=fixdt(1, 16)  OutScaling=2^0
  Divide : Product  Inputs=*/  OutDataType=fixdt(1, 16)  OutScaling=2^-10
  Integrator : Integrator  ExternalReset=rising  InitialConditionSource=external
  InvTauI : Gain  Gain=TauiInv  ParameterDataType=fixdt(1, 16)  ParameterScaling=2^0  OutDataType=fixdt(1, 16)  OutScaling=2^0
  Kp : Gain  Gain=Kp  ParameterDataType=fixdt(1, 16)  ParameterScaling=2^0  OutDataType=fixdt(1, 16)  OutScaling=2^0
  Saturation : Saturate  UpperLimit=UB  LowerLimit=LB  LinearizeAsGain=off  OutDataType=SaturationOutDataTypeStr
  Sum : Sum  Inputs=+-  OutDataType=fixdt(1, 16)  OutScaling=2^0
  Sum1 : Sum  Inputs=++|  OutDataType=fixdt(1, 16)  OutScaling=2^0
  Out1 : Outport
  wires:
  InvTauI/1 -> Integrator/1
  Sum1/1 -> Kp/1
  Integrator/1 -> Sum1/2
  Kp/1 -> Saturation/1
  In2/1 -> Integrator/2  "reset"
  In1/1 -> InvTauI/1, Sum1/1, Sum/2  "e"
  Saturation/1 -> Out1/1
  In3/1 -> Divide/1  "CV"
  Constant/1 -> Divide/2
  Divide/1 -> Sum/1
  Sum/1 -> Integrator/3

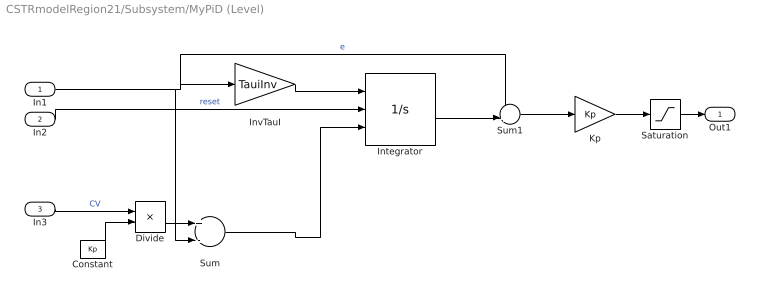
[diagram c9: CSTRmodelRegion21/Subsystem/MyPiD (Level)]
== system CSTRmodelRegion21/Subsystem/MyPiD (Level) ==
  In1 : Inport
  In2 : Inport  Port=2
  In3 : Inport  Port=3
  Constant : Constant  Value=Kp  OutDataType=fixdt(1, 16)  OutScaling=2^0
  Divide : Product  Inputs=*/  OutDataType=fixdt(1, 16)  OutScaling=2^-10
  Integrator : Integrator  ExternalReset=rising  InitialConditionSource=external
  InvTauI : Gain  Gain=TauiInv  ParameterDataType=fixdt(1, 16)  ParameterScaling=2^0  OutDataType=fixdt(1, 16)  OutScaling=2^0
  Kp : Gain  Gain=Kp  ParameterDataType=fixdt(1, 16)  ParameterScaling=2^0  OutDataType=fixdt(1, 16)  OutScaling=2^0
  Saturation : Saturate  UpperLimit=UB  LowerLimit=LB  LinearizeAsGain=off  OutDataType=SaturationOutDataTypeStr
  Sum : Sum  Inputs=+-  OutDataType=fixdt(1, 16)  OutScaling=2^0
  Sum1 : Sum  Inputs=++|  OutDataType=fixdt(1, 16)  OutScaling=2^0
  Out1 : Outport
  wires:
  InvTauI/1 -> Integrator/1
  Sum1/1 -> Kp/1
  Integrator/1 -> Sum1/2
  Kp/1 -> Saturation/1
  In2/1 -> Integrator/2  "reset"
  In1/1 -> InvTauI/1, Sum1/1, Sum/2  "e"
  Saturation/1 -> Out1/1
  In3/1 -> Divide/1  "CV"
  Constant/1 -> Divide/2
  Divide/1 -> Sum/1
  Sum/1 -> Integrator/3

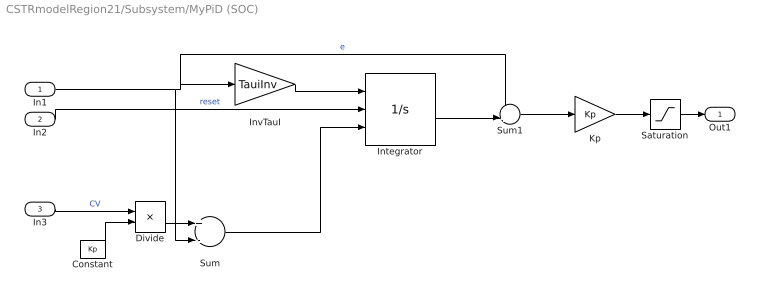
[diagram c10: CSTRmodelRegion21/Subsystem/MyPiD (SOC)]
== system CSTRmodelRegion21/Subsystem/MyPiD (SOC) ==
  In1 : Inport
  In2 : Inport  Port=2
  In3 : Inport  Port=3
  Constant : Constant  Value=Kp  OutDataType=fixdt(1, 16)  OutScaling=2^0
  Divide : Product  Inputs=*/  OutDataType=fixdt(1, 16)  OutScaling=2^-10
  Integrator : Integrator  ExternalReset=rising  InitialConditionSource=external
  InvTauI : Gain  Gain=TauiInv  ParameterDataType=fixdt(1, 16)  ParameterScaling=2^0  OutDataType=fixdt(1, 16)  OutScaling=2^0
  Kp : Gain  Gain=Kp  ParameterDataType=fixdt(1, 16)  ParameterScaling=2^0  OutDataType=fixdt(1, 16)  OutScaling=2^0
  Saturation : Saturate  UpperLimit=UB  LowerLimit=LB  LinearizeAsGain=off  OutDataType=SaturationOutDataTypeStr
  Sum : Sum  Inputs=+-  OutDataType=fixdt(1, 16)  OutScaling=2^0
  Sum1 : Sum  Inputs=++|  OutDataType=fixdt(1, 16)  OutScaling=2^0
  Out1 : Outport
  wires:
  InvTauI/1 -> Integrator/1
  Sum1/1 -> Kp/1
  Integrator/1 -> Sum1/2
  Kp/1 -> Saturation/1
  In2/1 -> Integrator/2  "reset"
  In1/1 -> InvTauI/1, Sum1/1, Sum/2  "e"
  Saturation/1 -> Out1/1
  In3/1 -> Divide/1  "CV"
  Constant/1 -> Divide/2
  Divide/1 -> Sum/1
  Sum/1 -> Integrator/3

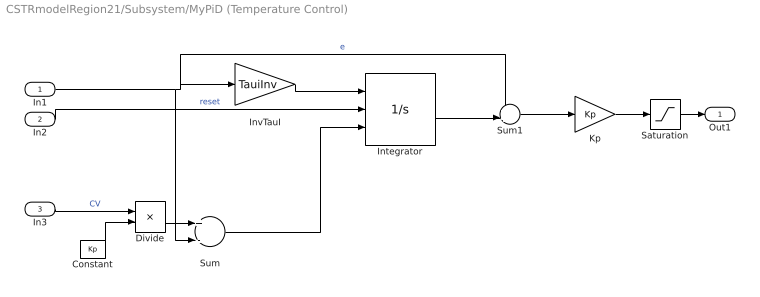
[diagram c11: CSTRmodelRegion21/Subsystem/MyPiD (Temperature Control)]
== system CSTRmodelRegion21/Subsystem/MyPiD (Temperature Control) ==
  In1 : Inport
  In2 : Inport  Port=2
  In3 : Inport  Port=3
  Constant : Constant  Value=Kp  OutDataType=fixdt(1, 16)  OutScaling=2^0
  Divide : Product  Inputs=*/  OutDataType=fixdt(1, 16)  OutScaling=2^-10
  Integrator : Integrator  ExternalReset=rising  InitialConditionSource=external
  InvTauI : Gain  Gain=TauiInv  ParameterDataType=fixdt(1, 16)  ParameterScaling=2^0  OutDataType=fixdt(1, 16)  OutScaling=2^0
  Kp : Gain  Gain=Kp  ParameterDataType=fixdt(1, 16)  ParameterScaling=2^0  OutDataType=fixdt(1, 16)  OutScaling=2^0
  Saturation : Saturate  UpperLimit=UB  LowerLimit=LB  LinearizeAsGain=off  OutDataType=SaturationOutDataTypeStr
  Sum : Sum  Inputs=+-  OutDataType=fixdt(1, 16)  OutScaling=2^0
  Sum1 : Sum  Inputs=++|  OutDataType=fixdt(1, 16)  OutScaling=2^0
  Out1 : Outport
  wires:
  InvTauI/1 -> Integrator/1
  Sum1/1 -> Kp/1
  Integrator/1 -> Sum1/2
  Kp/1 -> Saturation/1
  In2/1 -> Integrator/2  "reset"
  In1/1 -> InvTauI/1, Sum1/1, Sum/2  "e"
  Saturation/1 -> Out1/1
  In3/1 -> Divide/1  "CV"
  Constant/1 -> Divide/2
  Divide/1 -> Sum/1
  Sum/1 -> Integrator/3

== matlab function Self-optimizing 
Variable Region 1 ==
function cs = SOCVariable1(Fa,Fb,V,cVector)


cain        =  2;
cbin        = 1.5;
Fmax        = 22;
k2          =  0.0140;
cb          =  cVector(2);

cs = (-cbin^2*Fa^2-Fa^2*cain*cbin+6*Fa*cain*k2*cb^2*V+2*Fa*cain*Fmax*cb-Fa*cain*Fmax*cbin+4*V*k2*cb^3*Fmax+4*V^2*k2^2*cb^4-2*cbin*Fmax^2*cb+Fmax^2*cb^2-4*V*k2*cb^2*cbin*Fmax+cbin^2*Fmax^2);
%cs =cs/V;

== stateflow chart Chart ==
  state Region2/
    entry: 	R = 2;
    entry:	reset =1;
    during: 	R=2;
    during: 	reset=0;
  state Region1/
    entry: 	R =1;
    entry: 	reset =1;
    during: 	R=1;
    during: 	reset =0;
  state Region3/
    entry: 	R = 3;
    entry:	reset =1;
    during: 	R=3;
    during: 	reset=0;
  Region2 -> Region1 : [c1<0.001&]
  (default) -> Region3
  Region3 -> Region2 : [Ftot>=22]
